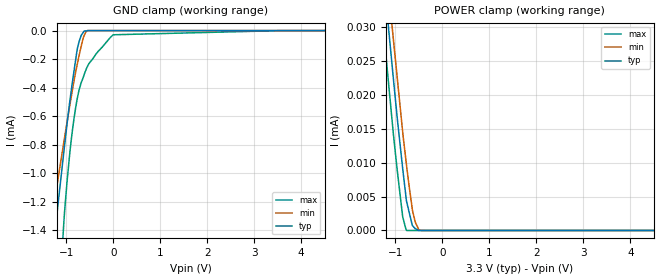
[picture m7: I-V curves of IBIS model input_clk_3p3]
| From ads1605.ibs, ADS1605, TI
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|   INPUT_CLK 3.3V Model
[Model]   input_clk_3p3
Model_type   Input
Vinl = 0.99
Vinh = 2.31
|   typ   min   max
|   (nom PVT)   (Fast PVT)   (Slow PVT)
C_comp   1.180e-12   1.160e-12   1.202e-12
|Where nom PVT is NOM Process, 3.3V,39C
|   Fast PVT is Strong Process, 3.6V, -40C
|   Slow PVT is Weak Process, 3.0V, 99C
[Model Spec]
Vinl   0.99   0.9   1.08
Vinh   2.31   2.1   2.52
[Voltage Range]   3.3   3   3.6
|Ambient Temperature   25   85   -40
|Junction Temperature
[Temperature Range]   39   99   -40
[Power Clamp Reference]   3.3   3   3.6
[GND Clamp Reference]   0   0   0
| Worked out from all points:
|   GND clamp passes 1 mA (typ) near -1.10 V on its own axis
[GND Clamp]
|   Voltage   I(typ)   I(min)   I(max)
-3.3V     -7.967mA   -5.703mA   -14.53mA
-1.36V    -1.779mA   -1.43mA    -3.029mA
-1.23V    -1.382mA   -1.152mA   -2.295mA
-1.136V   -1.099mA   -956.2uA   -1.787mA
-1.046V   -833.4uA   -769.5uA   -1.314mA
-927.6mV  -502.2uA   -529.5uA   -864.7uA
-834mV    -279.8uA   -347.3uA   -612.3uA
-729.3mV  -79.35uA   -177.3uA   -419uA
-617.1mV  -2.873uA   -33.46uA   -306.6uA
-517.2mV  0A         0A         -231.1uA
1.2mV     0A         0A         -29.3uA
6.6V      0A         0A         0A
[POWER Clamp]
|   Voltage   I(typ)   I(min)   I(max)
-3.3V     539.6uA    552.2uA    513.4uA
-2.022V   96.91uA    101.6uA    89.66uA
-1.241V   36.82uA    42.82uA    28.75uA
-1.162V   30.93uA    36.87uA    22.84uA
-1.074V   24.59uA    30.29uA    16.44uA
-1.043V   22.33uA    28.14uA    14.16uA
-848.4mV  9.323uA    14.72uA    2.212uA
-762.3mV  4.277uA    9.535uA    0A
-636mV    704.2nA    2.913uA    0A
-576mV    257.7nA    1.206uA    0A
-471.9mV  0A         16.03nA    0A
6.6V      0A         0A         0A
